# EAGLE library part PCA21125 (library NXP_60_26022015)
SPI-bus Real-Time Clock and calendar The PCA21125 is a CMOS1 Real-Time Clock (RTC) and calendar optimized for low-power consumption and an operating temperature up to 125 °C. Data is transferred via a Serial Peripheral Interface (SPI-bus) with a maximum data rate of 6.0 Mbit/s. Alarm and timer functions are also available with the possibility to generate a wake-up signal on the interrupt pin. AEC Q100 compliant for automotive applications. AAL Eindhoven MK
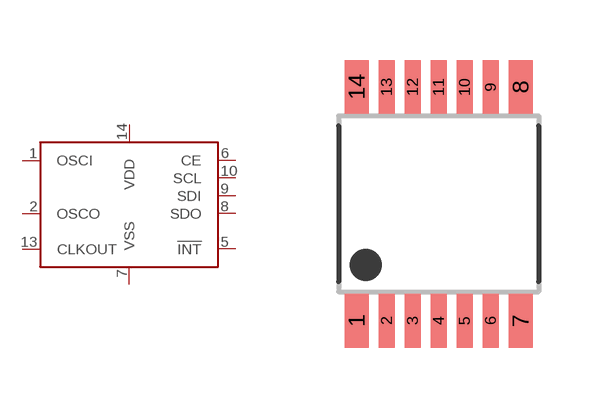
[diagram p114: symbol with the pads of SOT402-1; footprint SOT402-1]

Designator prefix U

## PCA21125T  [SOT402-1]
1  OSCI  pas
2  OSCO  pas
5  !INT  out
6  CE  in
7  VSS  pwr
8  SDO  out
9  SDI  in
10  SCL  in
13  CLKOUT  out
14  VDD  pwr

## Footprint SOT402-1 (pad centres in mm)
SOT402-1 TSSOP14: plastic thin shrink small outline package; 14 leads; body width 4.4 mm JEDEC: MO-153 IEC: ---
smd 0.6 x 1.35: 1 -2.05,-2.925; 7 2.05,-2.925; 8 2.05,2.925; 14 -2.05,2.925
smd 0.4 x 1.35: 2 -1.3,-2.925; 3 -0.65,-2.925; 4 0,-2.925; 5 0.65,-2.925; 6 1.3,-2.925; 9 1.3,2.925; 10 0.65,2.925; 11 0,2.925; 12 -0.65,2.925; 13 -1.3,2.925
